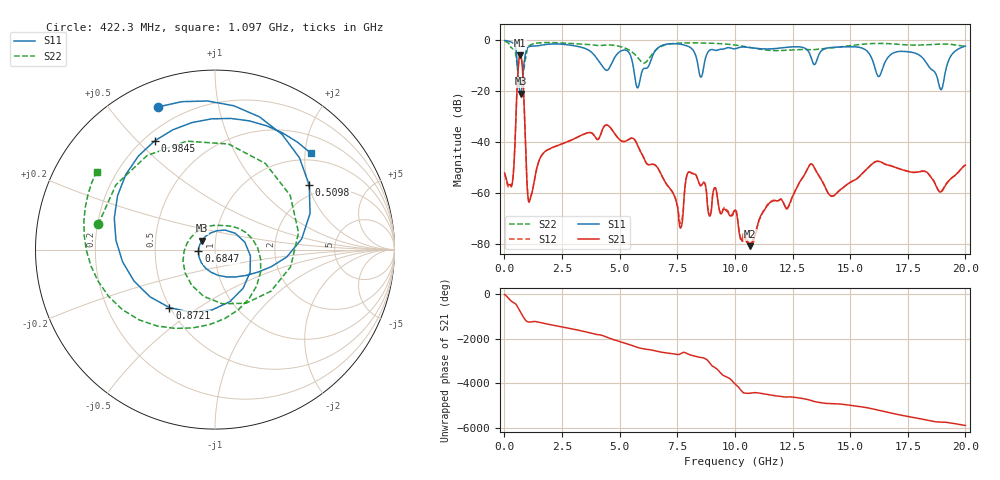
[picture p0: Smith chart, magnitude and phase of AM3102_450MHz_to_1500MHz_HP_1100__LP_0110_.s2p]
!Agilent Technologies,E8364B,MY43040894,A.07.50.67
!Agilent E8364B: A.07.50.67
!Date: Thursday, January 11, 2018 06:33:30
!Correction: S11(Full 2 Port(1,2))
!S21(Full 2 Port(1,2))
!S12(Full 2 Port(1,2))
!S22(Full 2 Port(1,2))
!S2P File: Measurements: S11, S21, S12, S22:
# Hz S  dB  R 50
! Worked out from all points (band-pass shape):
!   1601 points, 10 MHz to 20 GHz, reference 50 ohm
!   highest |S21| = -5.94 dB at 684.7 MHz (marker M1); lowest = -80.8 dB at 10.67 GHz (marker M2)
!   |S21| within 3 dB of the highest: 618.5 MHz to 765.7 MHz (147.2 MHz wide, 21.3 % of centre)
!   lowest |S11| = -21.0 dB at 709.6 MHz (marker M3), VSWR 1.20, Z = 43 + j4.39 ohm
!   |S11| at or under -10 dB: 5.585 GHz to 6.266 GHz (680.5 MHz wide, 11.5 % of centre); 16.05 GHz to 16.45 GHz (399.3 MHz wide, 2.46 % of centre); 18.38 GHz to 19.2 GHz (810.8 MHz wide, 4.32 % of centre)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
!   |S22| runs from -17.4 to -0.4 dB; largest |S21 - S12| = 0.00064
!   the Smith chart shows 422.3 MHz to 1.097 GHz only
!   S11 on the Smith chart (normalised r, x): 422.3 MHz: 0.11, +0.67; 509.8 MHz: 1.68, +2.03; 684.7 MHz: 0.83, -0.01; 872.1 MHz: 0.50, -0.38; 984.5 MHz: 0.24, +0.56; 1.097 GHz: 0.84, +2.12
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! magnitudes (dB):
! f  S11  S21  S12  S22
! 10 MHz  -0.1  -52.1  -52.5  -0.4
! 422.3 MHz  -1.4  -47.9  -47.4  -3.5
! 509.8 MHz  -3.9  -28.0  -28.0  -6.5
! 684.7 MHz  -20.6  -5.9  -5.9  -17.4
! 709.6 MHz  -21.0  -6.2  -6.2  -17.4
! 872.1 MHz  -7.7  -29.5  -29.6  -9.6
! 984.5 MHz  -3.2  -56.9  -56.3  -3.8
! 1.097 GHz  -2.4  -63.0  -62.4  -2.0
! 1.684 GHz  -1.8  -44.4  -44.4  -0.9
! 3.346 GHz  -2.8  -37.3  -37.3  -1.5
! 5.782 GHz  -18.7  -41.3  -41.3  -6.8
! 6.682 GHz  -2.8  -50.6  -50.5  -3.1
! 7.644 GHz  -1.6  -73.8  -72.0  -1.1
! 8.031 GHz  -2.6  -51.8  -51.7  -1.0
! 8.531 GHz  -14.5  -57.2  -56.9  -1.1
! 10.01 GHz  -3.4  -66.7  -66.6  -1.9
! 10.67 GHz  -2.9  -80.8  -80.3  -2.9
! 13.34 GHz  -7.8  -48.6  -48.7  -3.8
! 14.23 GHz  -2.8  -61.0  -61.2  -3.0
! 16.68 GHz  -6.4  -49.1  -49.1  -1.3
! 18.94 GHz  -19.4  -59.5  -59.4  -1.5
! 20 GHz  -2.3  -49.0  -49.0  -2.4
